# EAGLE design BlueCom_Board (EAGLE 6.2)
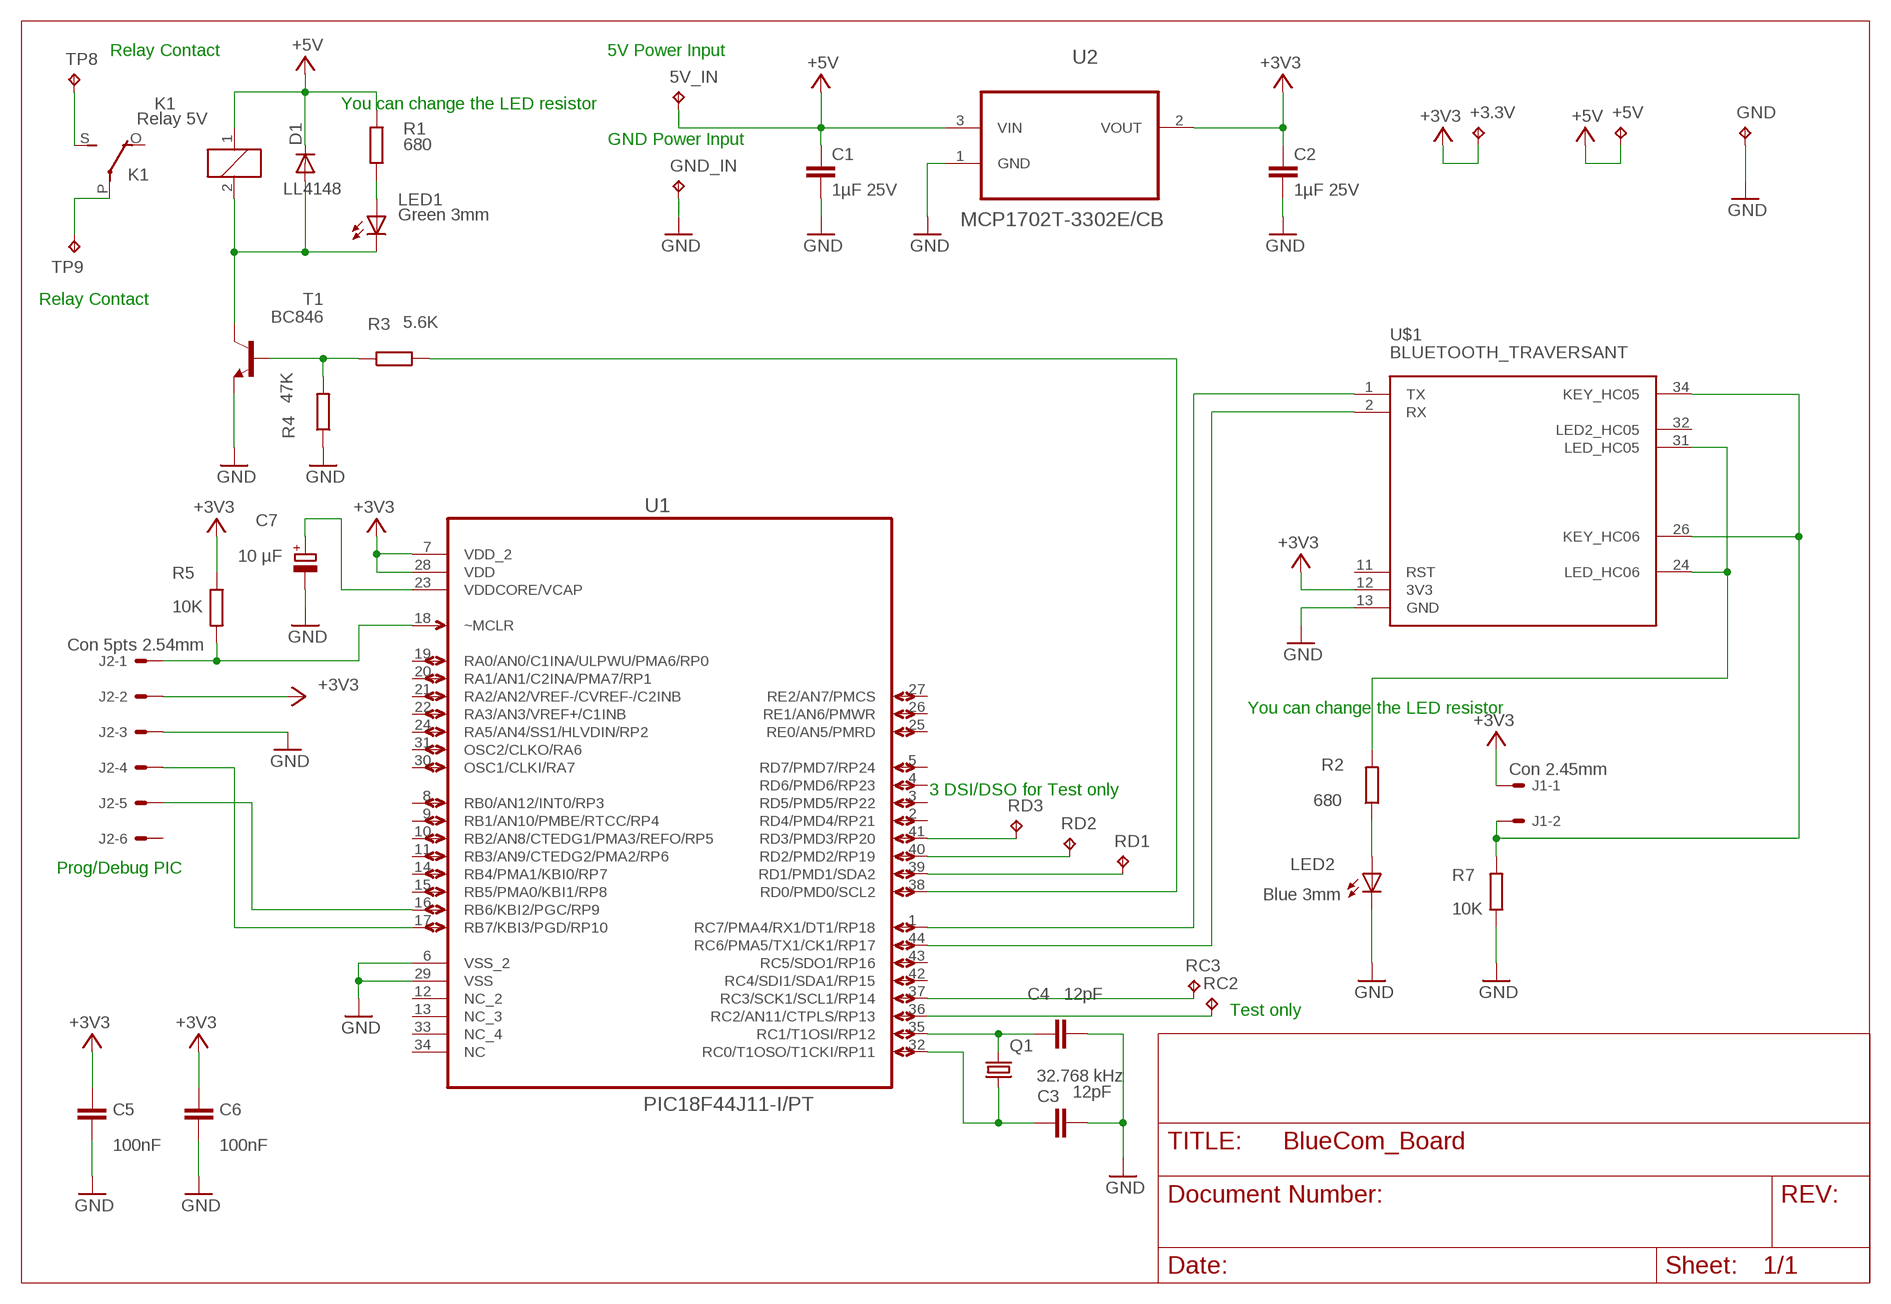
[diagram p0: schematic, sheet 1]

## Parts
5V_IN  TPPAD1-13Y  [P1-13Y]
+3.3V  TPPAD1-13  [P1-13]
+5V  TPPAD1-13  [P1-13]
C1  1µF 25V  C-EUC0805  [C0805]
C2  1µF 25V  C-EUC0805  [C0805]
C3  12pF  C-EUC0805  [C0805]
C4  12pF  C-EUC0805  [C0805]
C5  100nF  C-EUC0805  [C0805]
C6  100nF  C-EUC0805  [C0805]
C7  10 µF  CPOL-EUA/3216-18W  [A/3216-18W]
D1  LL4148  PMLL41SOD80C  [SOD80C]
GND  TPPAD1-13  [P1-13]
GND_IN  TPPAD1-13Y  [P1-13Y]
J1  Con 2.45mm  22-27-2021-02  [6410-02]
J2  Con 5pts 2.54mm  22-27-2061-06  [6410-06]
K1  Relay 5V  ZF112  [ZF112]
LED1  Green 3mm  LED3MM  [LED3MM]
LED2  Blue 3mm  LED3MM  [LED3MM]
Q1  32.768 kHz  CRYSTALTC26H  [TC26H]
R1  680  R-EU_R0805  [R0805]
R2  680  R-EU_R0805  [R0805]
R3  5.6K  R-EU_R0805  [R0805]
R4  47K  R-EU_R0805  [R0805]
R5  10K  R-EU_R0805  [R0805]
R7  10K  R-EU_R0805  [R0805]
RC2  TPPAD1-13  [P1-13]
RC3  TPPAD1-13  [P1-13]
RD1  TPPAD1-13  [P1-13]
RD2  TPPAD1-13  [P1-13]
RD3  TPPAD1-13  [P1-13]
T1  BC846  [SOT23]
TP8  TPPAD1-13Y  TPPAD1-20Y  [P1-20Y]
TP9  TPPAD1-13Y  TPPAD1-20Y  [P1-20Y]
U1  PIC18F44J11-I/PT  [QFP80P1200X1200X120-44N]
U2  MCP1702T-3302E/CB  [SOT95P255X145-3N]
U$1  BLUETOOTH_TRAVERSANT  [BLUETOOTH_TRAVERSANT]

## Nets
+3V3: +3.3V.TP C2.1 C5.1 C6.1 J1.1 J2.2 R5.1 U1.7(VDD_2) U1.28(VDD) U2.2(VOUT) U$1.12(3V3)
+5V: 5V_IN.TP +5V.TP C1.1 D1.C K1.1 R1.2 U2.3(VIN)
GND: C1.2 C2.2 C3.2 C4.2 C5.2 C6.2 C7.- GND.TP GND_IN.TP J2.3 LED2.K(C) R4.1 R7.1 T1.2(E) U1.6(VSS_2) U1.29(VSS) U2.1(GND) U$1.13(GND)
N$1: D1.A K1.2 LED1.K(C) T1.3(C)
N$2: R3.1 R4.2 T1.1(B)
N$3: RD3.TP U1.41(RD3/PMD3/RP20)
N$4: LED1.A R1.1
N$5: LED2.A R2.1
N$6: R2.2 U$1.24(LED_HC06) U$1.31(LED_HC05)
N$7: J1.2 R7.2 U$1.26(KEY_HC06) U$1.34(KEY_HC05)
N$8: U1.44(RC6/PMA5/TX1/CK1/RP17) U$1.2(RX)
N$9: U1.1(RC7/PMA4/RX1/DT1/RP18) U$1.1(TX)
N$10: K1.S(2:S) TP8.TP
N$11: K1.P(2:P) TP9.TP
N$12: J2.1 R5.2 U1.18(~MCLR)
N$13: C4.1 Q1.2 U1.35(RC1/T1OSI/RP12)
N$14: C3.1 Q1.1 U1.32(RC0/T1OSO/T1CKI/RP11)
N$15: J2.5 U1.16(RB6/KBI2/PGC/RP9)
N$16: RD2.TP U1.40(RD2/PMD2/RP19)
N$17: C7.+ U1.23(VDDCORE/VCAP)
N$18: R3.2 U1.38(RD0/PMD0/SCL2)
N$19: J2.4 U1.17(RB7/KBI3/PGD/RP10)
N$20: RD1.TP U1.39(RD1/PMD1/SDA2)
N$21: RC2.TP U1.36(RC2/AN11/CTPLS/RP13)
N$22: RC3.TP U1.37(RC3/SCK1/SCL1/RP14)
Unconnected: J2.6 K1.O(2:O) U1.2(RD4/PMD4/RP21) U1.3(RD5/PMD5/RP22) U1.4(RD6/PMD6/RP23) U1.5(RD7/PMD7/RP24) U1.8(RB0/AN12/INT0/RP3) U1.9(RB1/AN10/PMBE/RTCC/RP4) U1.10(RB2/AN8/CTEDG1/PMA3/REFO/RP5) U1.11(RB3/AN9/CTEDG2/PMA2/RP6) U1.12(NC_2) U1.13(NC_3) U1.14(RB4/PMA1/KBI0/RP7) U1.15(RB5/PMA0/KBI1/RP8) U1.19(RA0/AN0/C1INA/ULPWU/PMA6/RP0) U1.20(RA1/AN1/C2INA/PMA7/RP1) U1.21(RA2/AN2/VREF-/CVREF-/C2INB) U1.22(RA3/AN3/VREF+/C1INB) U1.24(RA5/AN4/SS1/HLVDIN/RP2) U1.25(RE0/AN5/PMRD) U1.26(RE1/AN6/PMWR) U1.27(RE2/AN7/PMCS) U1.30(OSC1/CLKI/RA7) U1.31(OSC2/CLKO/RA6) U1.33(NC_4) U1.34(NC) U1.42(RC4/SDI1/SDA1/RP15) U1.43(RC5/SDO1/RP16) U$1.11(RST) U$1.32(LED2_HC05)

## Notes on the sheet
- Relay Contact | 5V Power Input
- You can change the LED resistor
- GND Power Input
- Relay Contact
- You can change the LED resistor
- 3 DSI/DSO for Test only
- Prog/Debug PIC
- Test only

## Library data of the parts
5V_IN +3.3V +5V GND GND_IN RC2 RC3 RD1-RD3 TP8 TP9 = testpad:TP: Test pad
C1-C6 = rcl:C-EU: CAPACITOR, European symbol
C7 = rcl:CPOL-EU: POLARIZED CAPACITOR, European symbol
D1 = diode:PMLL41*: High-speed diodes
J1 = con-molex:22-?-02: CONNECTOR; OC_FARNELL: unknown; OC_NEWARK: unknown
J2 = con-molex:22-?-06: CONNECTOR wire to board 2.54 mm (.1 inch) pitch header; OC_FARNELL: unknown; OC_NEWARK: unknown
K1 = relay:ZF112: RELAY 1 x switch; OC_FARNELL: unknown; OC_NEWARK: unknown
LED1 LED2 = led:LED: LED
Q1 = crystal:CRYSTAL: CRYSTAL; OC_FARNELL: unknown; OC_NEWARK: unknown
R1-R5 R7 = resistor:R-EU_: RESISTOR, European symbol
T1 = transistor:BC846: NPN TRANSISTOR
U1 = BlueCom_Lib:PIC18F44J11-I/PT: High-Performance Microcontrollers; DESCRIPTION: 8BIT MCU; MPN: pic18f44j11-I/pt; OC_FARNELL: 1702900; OC_NEWARK: 98M1811; PACKAGE: TQFP-44; SUPPLIER: Microchip
U2 = BlueCom_Lib:MCP1702T-3302E/CB: 250 mA Low Quiescent Current LDO Regulator; MPN: MCP1702T-3302E/CB; OC_FARNELL: 1331490; OC_NEWARK: 84R5179; PACKAGE: SOT23-3; SUPPLIER: Microchip
U$1 = BlueCom_Lib:BLUETOOTH_TRAVERSANT

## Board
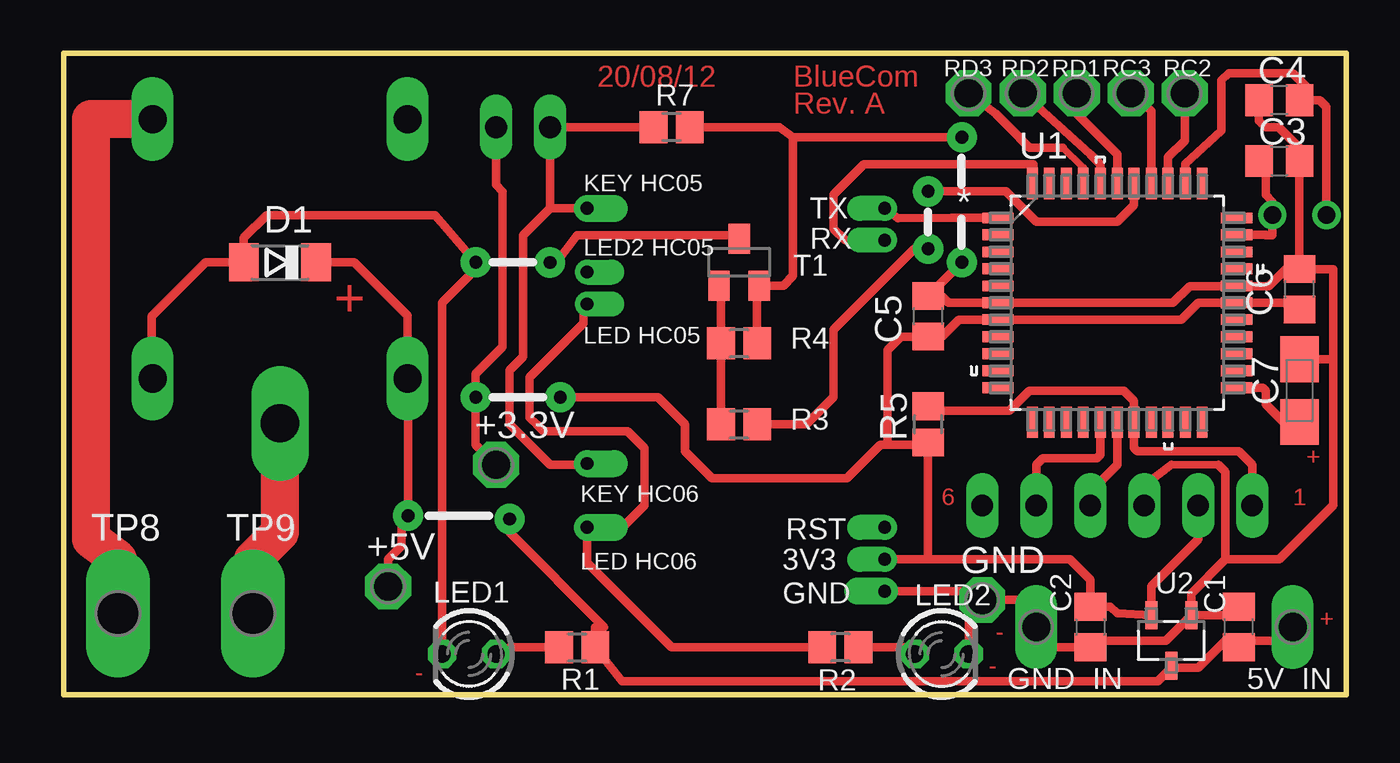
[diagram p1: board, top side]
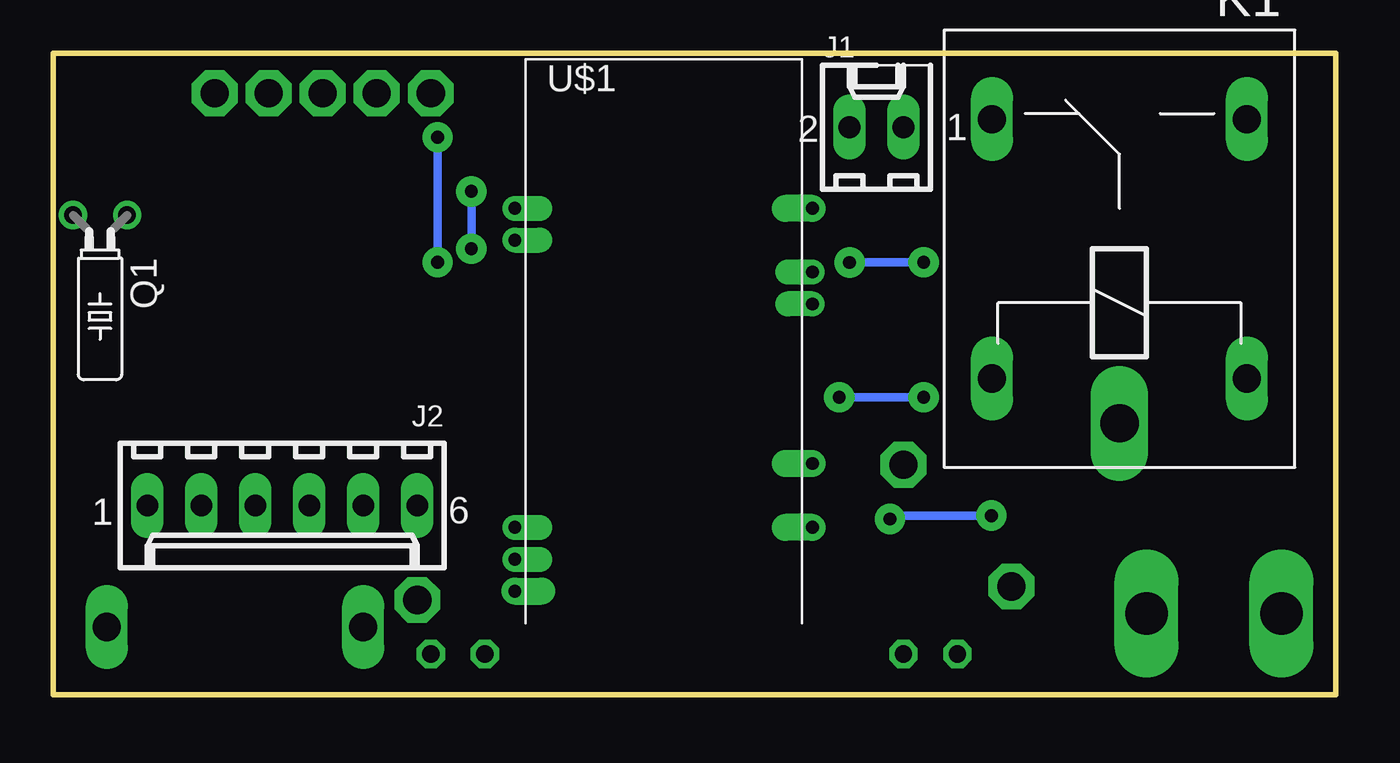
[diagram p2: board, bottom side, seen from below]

Size 60.3 x 30.15 mm. Coordinates in mm from the lower left corner, seen from the top.
Outline: 0,0 60.3,0 60.3,30.15 0,30.15 0,0
Copper layers (1*16): Top 0.035mm / dielectric 1.5mm / Bottom 0.035mm
Design rules: minimum track width 10mil, minimum drill 24mil, track to track 8mil, track to pad 8mil, pad to pad 8mil, via to via 8mil, smd to smd 8mil, copper to edge 0.5mm, drill to drill 6mil, minimum pad ring 10mil, minimum via ring 8mil, stop-mask expansion 4mil, vias tented up to drill 0mil, thermal gap 10mil

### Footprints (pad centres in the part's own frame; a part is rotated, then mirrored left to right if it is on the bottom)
P1-13Y = drill 1.321 pad 1.905 long: TP 0,0
P1-13 = drill 1.321 pad 2.159 octagon: TP 0,0
C0805 = smd 1.3 x 1.5: 1 -0.95,0; 2 0.95,0
A/3216-18W = smd 2.15 x 1.8: + 1.475,0; - -1.475,0
SOD80C = smd 1.4 x 1.8: A 1.7,0; C -1.7,0
6410-02 = drill 1.016 long: 1 1.27,0; 2 -1.27,0
6410-06 = drill 1.016 long: 1 6.35,0; 2 3.81,0; 3 1.27,0; 4 -1.27,0; 5 -3.81,0; 6 -6.35,0
ZF112 = drill 1.321 long: 1 -6.096,5.994; 2 -6.096,-5.994; O 6.096,5.994; S 6.096,-5.994 | drill 1.803 long: P -8.204,0
LED3MM = drill 0.813 octagon: A -1.27,0; K 1.27,0
TC26H = drill 0.813: 1 -1.27,0; 2 1.27,0
R0805 = smd 1.3 x 1.5: 1 -0.85,0; 2 0.85,0
SOT23 = smd 1 x 1.4: 1 -0.95,-1.1; 2 0.95,-1.1; 3 0,1.1
P1-20Y = drill 2.007 pad 2.54 long: TP 0,0
QFP80P1200X1200X120-44N = smd 1.473 x 0.508: 1 -5.613,3.988; 2 -5.613,3.2; 3 -5.613,2.388; 4 -5.613,1.6; 5 -5.613,0.787; 6 -5.613,0; 7 -5.613,-0.787; 8 -5.613,-1.6; 9 -5.613,-2.388; 10 -5.613,-3.2; 11 -5.613,-3.988; 23 5.613,-3.988; 24 5.613,-3.2; 25 5.613,-2.388; 26 5.613,-1.6; 27 5.613,-0.787; 28 5.613,0; 29 5.613,0.787; 30 5.613,1.6; 31 5.613,2.388; 32 5.613,3.2; 33 5.613,3.988 | smd 0.508 x 1.473: 12 -3.988,-5.613; 13 -3.2,-5.613; 14 -2.388,-5.613; 15 -1.6,-5.613; 16 -0.787,-5.613; 17 0,-5.613; 18 0.787,-5.613; 19 1.6,-5.613; 20 2.388,-5.613; 21 3.2,-5.613; 22 3.988,-5.613; 34 3.988,5.613; 35 3.2,5.613; 36 2.388,5.613; 37 1.6,5.613; 38 0.787,5.613; 39 0,5.613; 40 -0.787,5.613; 41 -1.6,5.613; 42 -2.388,5.613; 43 -3.2,5.613; 44 -3.988,5.613
SOT95P255X145-3N = smd 0.559 x 1.321: 1 -0.94,-1.194; 2 0.94,-1.194; 3 0,1.194
BLUETOOTH_TRAVERSANT = drill 0.6 pad 1.17 offset: 1 -0.5,0; 2 -0.5,-1.5; 11 -0.5,-15; 12 -0.5,-16.5; 31 13.5,-4.5; 32 13.5,-3 | drill 0.6 pad 1.27 offset: 13 -0.5,-18; 24 13.5,-15; 26 13.5,-12; 34 13.5,0

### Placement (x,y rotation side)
5V_IN  57.78,3.17 0 top
+3.3V  20.32,10.79 0 top
+5V  15.24,5.08 0 top
C1  55.24,3.17 90 top
C2  48.26,3.17 270 top
C3  57.15,25.08 0 top
C4  57.15,27.94 180 top
C5  40.64,17.78 90 top
C6  58.1,19.05 90 top
C7  58.1,14.29 270 top
D1  10.16,20.32 180 top
GND  43.18,4.45 0 top
GND_IN  45.72,3.17 0 top
J1  21.59,26.67 0 bottom
J2  49.53,8.89 180 bottom
K1  10.16,20.95 90 bottom
LED1  19.05,1.91 180 top
LED2  41.27,1.91 0 top
Q1  58.1,22.54 180 bottom
R1  24.13,2.22 0 top
R2  36.51,2.22 180 top
R3  31.75,12.7 0 top
R4  31.75,16.51 180 top
R5  40.64,12.7 90 top
R7  28.57,26.67 180 top
RC2  52.71,28.26 0 top
RC3  50.17,28.26 0 top
RD1  47.62,28.26 0 top
RD2  45.09,28.26 0 top
RD3  42.55,28.26 0 top
T1  31.75,20.32 0 top
TP8  2.54,3.81 0 top
TP9  8.89,3.81 0 top
U1  49.53,18.41 0 top
U2  52.07,2.54 180 top
U$1  38.1,22.86 0 bottom

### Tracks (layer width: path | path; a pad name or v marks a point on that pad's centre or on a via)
+3V3  (via drill 0.6 pad 1.42)
  Top 0.406: C6.1 58.1,18.41 U1.28 53.34,18.41 52.55,17.63 U1.7 42.08,17.63 41.27,16.83 C5.1 | J2.2 53.34,7.3 51.13,5.09 U2.2 49.53,3.81 49.21,4.13 C2.1 48.26,5.4 47.31,6.35 40.64,6.35 | C5.1 | C5.1 39.37,16.83 38.73,16.19 38.73,11.75 40.01,11.75 | 40.01,11.75 40.54,11.75 R5.1 40.64,6.35 | 40.64,6.35 U$1.12 | v23.34,13.97 27.94,13.97 29.21,12.7 29.21,11.43 30.48,10.16 36.82,10.16 38.41,11.74 40,11.74 40.01,11.75 | J1.1 20.32,23.96 20.63,23.65 20.63,16.35 19.36,15.08 v19.36,13.98 | v19.36,13.98 v19.37,13.97 | v19.36,13.98 19.36,11.75 +3.3V.TP
  Bottom 0.406: v19.37,13.97 v23.34,13.97
+5V  (via drill 0.6 pad 1.42)
  Top 0.406: 52.07,1.27 53.34,1.27 54.61,2.54 C1.1 55.88,2.54 57.15,2.54 5V_IN.TP | 52.07,1.27 U2.3 | D1.C 13.65,20.32 16.15,17.82 K1.1 16.19,14.83 v16.19,8.41 15.88,8.1 15.88,6.99 15.24,6.35 +5V.TP | 52.07,1.27 51.44,0.64 26.25,0.64 R1.2 24.98,3.17 25.4,3.17 20.95,7.62 v20.95,8.26
  Bottom 0.406: v16.19,8.41 20.8,8.41 v20.95,8.26
GND  (via drill 0.6 pad 1.42)
  Top 0.356: 54.29,10.79 52.07,10.79
  Top 0.406: C6.2 57.47,20 56.67,19.2 U1.29 52.94,19.2 52.15,18.41 U1.6 41.59,18.41 41.27,18.73 C5.2 v42.23,20.32 | 58.42,20 C6.2 | U2.1 51.82,2.54 48.26,2.54 C2.2 46.35,2.22 45.72,2.86 GND_IN.TP 45.72,4.45 GND.TP | U2.1 54.85,3.73 C1.2 | U2.1 53.01,4.75 54.61,6.35 | 54.61,6.35 54.61,10.48 54.29,10.79 | 52.07,10.79 50.8,9.84 J2.3 | 59.17,15.76 C7.- 59.69,15.76 | 59.69,15.76 59.69,8.89 57.15,6.35 54.61,6.35 | 59.69,15.76 59.69,20 58.42,20 | 58.42,20 C6.2 | C6.2 | v42.23,26.19 34.29,26.19 | R4.1 32.6,19.12 T1.2 33.83,19.22 34.29,19.68 34.29,26.19 | C4.2 56.2,26.98 56.52,26.67 57.12,26.67 58.08,25.71 58.08,25.1 C3.2 C6.2 | R7.1 33.66,26.67 34.29,26.19 | U$1.13 42.77,4.86 GND.TP | LED2.K 42.55,3.81 GND.TP
  Bottom 0.406: v42.23,20.32 v42.23,26.19
N$1  (via drill 0.6 pad 1.42)
  Top 0.406: K1.2 4.13,14.86 4.13,17.78 6.67,20.32 D1.A 8.46,21.48 9.53,22.54 17.46,22.54 v19.37,20.32 19.37,20 17.77,18.41 LED1.K | v22.85,20.31 23.17,20.31 24.13,21.59 31.58,21.59 T1.3
  Bottom 0.406: v19.37,20.32 22.53,20.32 v22.85,20.31
N$2
  Top 0.406: R3.1 R4.2 30.9,19.12 T1.1
N$3
  Top 0.33: 47.93,24.75 46.98,25.71
  Top 0.356: U1.41 47.93,24.75
  Top 0.406: 46.98,25.71 45.41,25.71 44.45,26.67 43.81,27.3 RD3.TP
N$4
  Top 0.406: LED1.A 20.95,2.22 R1.1
N$5
  Top 0.406: LED2.A 39.69,2.22 R2.1
N$6
  Top 0.406: 24.65,18.31 U$1.31 24.44,18.2 24.44,17.46 22.86,15.88 21.9,14.92 21.9,13.01 22.21,12.7 22.23,12.7 22.55,12.38 26.5,12.38 27.3,11.58 27.3,8.89 26.27,7.86 U$1.24 24.6,6.19 28.57,2.22 R2.2
N$7
  Top 0.406: R7.2 J1.2 22.86,22.86 | U$1.34 22.86,22.86 | 22.86,22.86 21.59,21.59 21.59,15.88 20.95,15.24 20.95,12.7 22.86,10.79 24.54,10.79 U$1.26
N$8
  Top 0.406: U$1.2 36.74,21.36 36.2,21.91 36.2,23.5 37.62,24.92 45.6,24.92 U1.44
N$9
  Top 0.406: U1.1 41.73,22.4 39.21,22.38 U$1.1
N$10
  Top 1.27: 2.54,6.35 TP8.TP
  Top 1.778: K1.S 1.27,27.05 1.27,7.3 2.54,6.35
N$11
  Top 1.27: TP9.TP 8.89,6.35
  Top 1.778: 8.89,6.35 10.16,7.62 K1.P
N$12
  Top 0.406: J2.1 55.88,10.79 55.24,11.43 50.48,11.43 50.32,11.6 U1.18 50.32,13.82 49.85,14.29 45.4,14.29 44.45,13.34 40.85,13.34 R5.2
N$13
  Top 0.406: U1.35 52.73,24.96 54.43,26.5 54.43,28.88 54.77,29.21 57.78,29.21 58.42,28.57 58.42,28.26 C4.1 59.05,27.94 59.37,27.62 Q1.2
N$14
  Top 0.406: C3.1 56.52,24.77 56.52,23.5 56.83,23.18 Q1.1 56.83,21.59 56.52,21.59 56.52,21.61 U1.32
N$15
  Top 0.406: U1.16 48.74,11.28 48.58,11.11 46.04,11.11 45.72,10.79 J2.5
N$16
  Top 0.406: U1.40 48.74,24.92 48.26,25.4 | 48.26,25.4 | 48.26,25.4 RD2.TP
N$17
  Top 0.406: U1.23 56.38,14.43 56.52,14.29 56.52,13.65 57.47,12.7 57.99,12.7 C7.+
N$18  (via drill 0.6 pad 1.42)
  Top 0.406: U1.38 50.32,23.01 49.53,22.23 45.72,22.23 44.29,23.65 v40.64,23.65 | v40.64,20.95 40.01,20.95 36.2,17.14 36.2,13.97 34.92,12.7 R3.2
  Bottom 0.406: v40.64,23.65 v40.64,20.95
N$19
  Top 0.406: U1.17 49.53,10.79 48.26,9.53 J2.4
N$20
  Top 0.406: U1.39 49.53,25.4 47.62,27.3 RD1.TP
N$21
  Top 0.406: U1.36 51.92,25.25 52.7,26.04 52.7,28.58 RC2.TP
N$22
  Top 0.406: U1.37 51.13,27.45 RC3.TP

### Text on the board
Top: 20/08/12 | BlueCom | Rev. A | + | + | 6 | 1 | - | + | - | -
tPlace: KEY HC05 | TX | LED2 HC05 | RX | LED HC05 | KEY HC06 | RST | LED HC06 | 3V3 | GND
